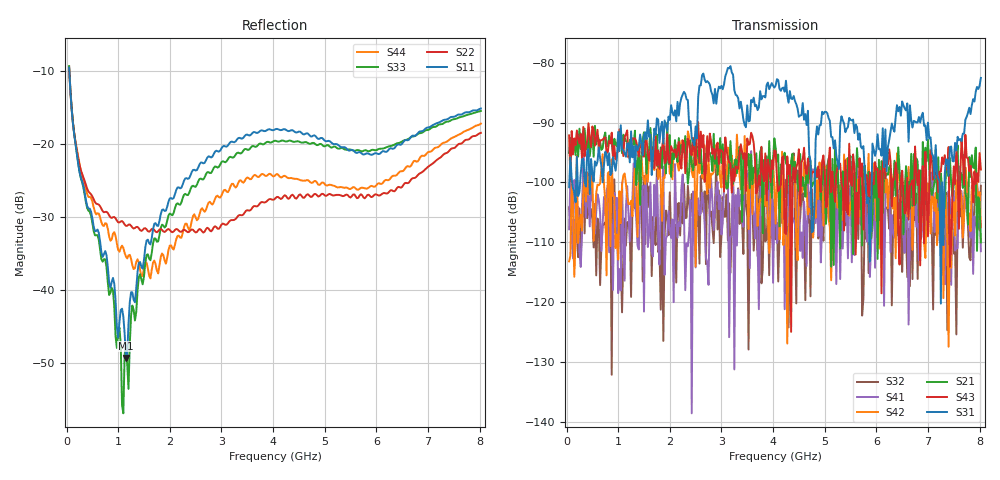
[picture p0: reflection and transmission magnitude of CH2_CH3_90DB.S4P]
!Agilent Technologies,E5071C,MY46316741,A.11.02
!Date: Thu May 28 14:48:18 2026
!Data & Calibration Information:
!1:CH2 INPUT 2:CH2 OUTPUT 3:CH3 INPUT 4:CH3 OUTPUT
!Freq	S11:SOLT4(ON)	S12:SOLT4(ON)	S13:SOLT4(ON)	S14:SOLT4(ON)
!	S21:SOLT4(ON)	S22:SOLT4(ON)	S23:SOLT4(ON)	S24:SOLT4(ON)
!	S31:SOLT4(ON)	S32:SOLT4(ON)	S33:SOLT4(ON)	S34:SOLT4(ON)
!	S41:SOLT4(ON)	S42:SOLT4(ON)	S43:SOLT4(ON)	S44:SOLT4(ON)
!PortZ  Port1:50+j0  Port2:50+j0  Port3:50+j0  Port4:50+j0
!Above PortZ is port z conversion or system Z0 setting when saving the data.
!When reading, reference impedance value at option line is always used.
# Hz S dB R 50
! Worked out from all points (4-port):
!   320 points, 50 MHz to 8.025 GHz, reference 50 ohm
!   strongest paths, dB at 50 MHz, 2.05 GHz, 4.05 GHz, 6.05 GHz, 8.025 GHz:
!     S31: -100.8, -88.3, -83.8, -94.4, -82.5
!     S43: -92.1, -94.6, -94.8, -102.5, -97.8
!     S21: -95.1, -95.1, -94.2, -96.2, -110.0
!     S42: -113.2, -99.5, -106.9, -111.1, -107.5
!     S41: -107.8, -106.2, -101.9, -102.4, -111.5
!     S32: -104.2, -108.2, -109.5, -107.8, -100.6
!   lowest |S11| = -49.4 dB at 1.15 GHz (marker M1), VSWR 1.01, Z = 49.9 - j0.322 ohm
!   |S11| at or under -10 dB: 53.66 MHz to end of sweep
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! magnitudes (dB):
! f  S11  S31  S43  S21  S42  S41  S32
! 50 MHz  -9.5  -100.8  -92.1  -95.1  -113.2  -107.8  -104.2
! 400 MHz  -28.5  -94.9  -93.0  -94.5  -98.3  -98.6  -106.0
! 1.1 GHz  -43.7  -94.7  -95.6  -92.0  -98.8  -109.9  -112.4
! 1.15 GHz  -49.4  -95.7  -92.0  -93.1  -100.2  -104.2  -110.6
! 1.55 GHz  -33.2  -92.8  -92.9  -98.5  -95.6  -101.8  -98.2
! 2.9 GHz  -20.9  -86.9  -94.5  -94.8  -97.0  -101.0  -96.4
! 8.025 GHz  -15.1  -82.5  -97.8  -110.0  -107.5  -111.5  -100.6
